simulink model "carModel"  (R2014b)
settings: Solver=ode3  StartTime=0.0  StopTime=10.0  FixedStep=.01  RelTol=1e-3
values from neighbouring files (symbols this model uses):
  A = [0 1;0 0]    [car.m]
  B = [0;1]    [car.m]
  C = [1 0]    [car.m]
  d = .2    (= 0.2)    [car.m]
  K = acker(A',C',poles)'    [car.m]
libraries: simulink x1

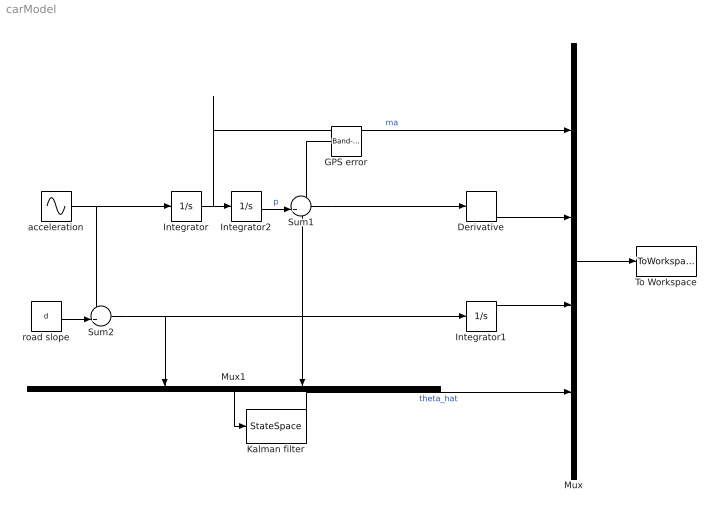
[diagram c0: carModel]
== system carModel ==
  Derivative : Derivative
  GPS error : simulink/Sources/Band-Limited White Noise  Cov=n  Ts=0.01  seed=[23341]
  Integrator : Integrator
  Integrator1 : Integrator
  Integrator2 : Integrator
  Kalman filter : StateSpace  A=A-K*C  B=[B K]  C=[0 1]  D=[0 0]  X0=0
  Mux : Mux
  Mux1 : Mux  Inputs=2
  Sum1 : Sum  Inputs=++|
  Sum2 : Sum  Inputs=++|
  To Workspace : ToWorkspace  VariableName=simout  SaveFormat=Timeseries  SampleTime=-1
  acceleration : Sin  SampleTime=0
  road slope : Constant  Value=d
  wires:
  Integrator/1 -> Integrator2/1, Mux/1  "ma"
  Integrator1/1 -> Mux/3
  Mux/1 -> To Workspace/1
  Derivative/1 -> Mux/2
  Mux1/1 -> Kalman filter/1
  Kalman filter/1 -> Mux/4  "theta_hat"
  GPS error/1 -> Sum1/1
  Sum1/1 -> Mux1/2, Derivative/1
  Integrator2/1 -> Sum1/2  "p"
  acceleration/1 -> Integrator/1, Sum2/1
  Sum2/1 -> Mux1/1, Integrator1/1
  road slope/1 -> Sum2/2
